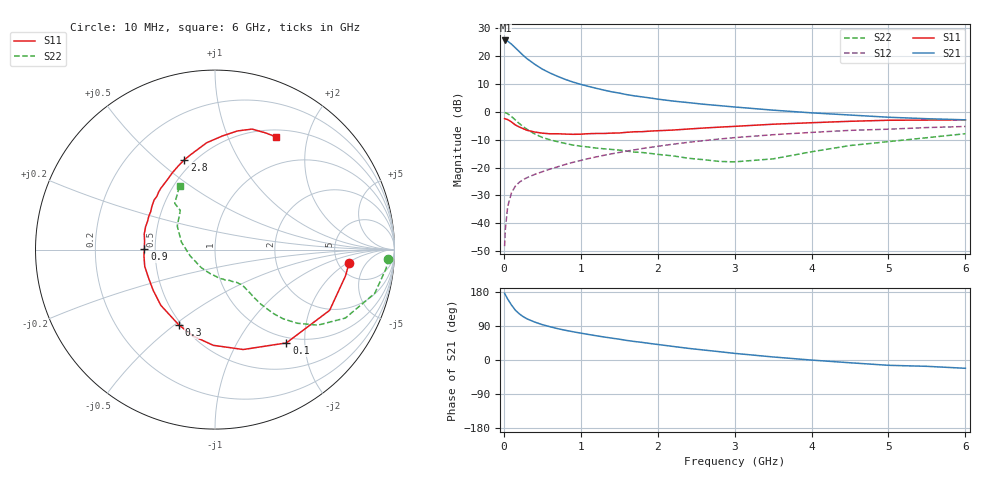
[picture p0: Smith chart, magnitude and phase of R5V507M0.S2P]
! SIEMENS Small Signal Semiconductors
! BFR183
! Si NPN RF Bipolar Junction Transistor in SOT23
! VCE = 0.5 V  IC = 7 mA
! Common Emitter S-Parameters:  May  1996
# GHz  S  MA  R  50
!  f  S11  S21  S12  S22
! GHz  MAG  ANG  MAG  ANG  MAG  ANG  MAG  ANG
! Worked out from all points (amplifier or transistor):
!   36 points, 10 MHz to 6 GHz, reference 50 ohm
!   highest |S21| = 25.5 dB at 20 MHz (marker M1)
!   |S21| within 3 dB of that: start of sweep to 163.3 MHz
!   unconditionally stable (mu >= 1): 762.3 MHz to 3.485 GHz
!   at 250 MHz: K = 0.54, MSG = 22.3 dB, |S12| = -24.3 dB
!   at 1.4 GHz: K = 1.11, MAG = 9.1 dB, |S12| = -15.1 dB
!   at 6 GHz: K = 0.98, MSG = 1.2 dB, |S12| = -5.3 dB
!   S11 on the Smith chart (normalised r, x): 10 MHz: 6.22, -2.20; 100 MHz: 0.90, -1.64; 300 MHz: 0.48, -0.52; 900 MHz: 0.44, +0.00; 2.8 GHz: 0.44, +0.62; 6 GHz: 0.59, +1.51
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0.01  0.7506 -5.9  18.84 176.3  0.0039 84.4  0.9662 -3.0
0.02  0.7414 -11.5  18.9 172.0  0.0079 82.6  0.9592 -6.3
0.05  0.7227 -27.9  18.38 160.8  0.02 77.4  0.9228 -15.3
0.1  0.6545 -52.6  16.2 144.9  0.0355 66.2  0.8205 -27.7
0.15  0.5785 -74.2  13.93 131.4  0.0465 59.0  0.711 -36.3
0.2  0.5335 -91.0  11.96 122.0  0.0543 55.2  0.6157 -41.8
0.25  0.4969 -104.2  10.25 114.6  0.0607 53.2  0.5418 -45.4
0.3  0.4651 -115.8  8.941 108.7  0.0657 52.1  0.4851 -47.5
0.4  0.433 -134.2  7.1 100.2  0.0752 52.1  0.4005 -49.9
0.5  0.4125 -146.6  5.795 93.3  0.0841 52.7  0.346 -50.8
0.6  0.4023 -157.8  4.937 87.8  0.0938 53.2  0.3141 -51.1
0.7  0.4024 -166.7  4.295 82.7  0.103 54.1  0.2897 -51.5
0.9  0.3935 179.3  3.393 74.5  0.124 55.1  0.2525 -52.3
1.1  0.4038 167.5  2.842 67.4  0.1445 55.1  0.2328 -54.8
1.3  0.4073 157.4  2.44 60.8  0.1654 54.4  0.2166 -57.1
1.6  0.4278 144.9  2.021 51.6  0.1971 52.6  0.1969 -63.0
2.2  0.469 125.1  1.551 35.8  0.2617 47.1  0.1616 -81.2
2.8  0.5288 108.8  1.286 22.0  0.324 40.0  0.1287 -113.4
3.5  0.5968 94.5  1.066 8.0  0.3871 30.5  0.143 -165.8
4.5  0.6732 79.2  0.872 -7.3  0.4633 17.2  0.2477 148.1
5.5  0.7084 66.7  0.749 -16.7  0.5199 6.0  0.3421 131.0
6  0.7139 61.8  0.715 -21.9  0.5439 -1.4  0.4038 119.3
